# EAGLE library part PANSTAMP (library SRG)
panStamp panStamps are small wireless modules programmable from the Arduino IDE. Each module contains an Atmega328p MCU and a Texas Instruments CC1101 RF interface, providing the necessary connectivity and processing power to create autonomous low-power wireless motes. Everything contained into a compact DIP-24 module. http://www.panstamp.com Vin: 2.5 to 3.6 volts A4 - SDA A5 - SCL PWM: D3,5,6,9,10,11 Interrupts: D2,3
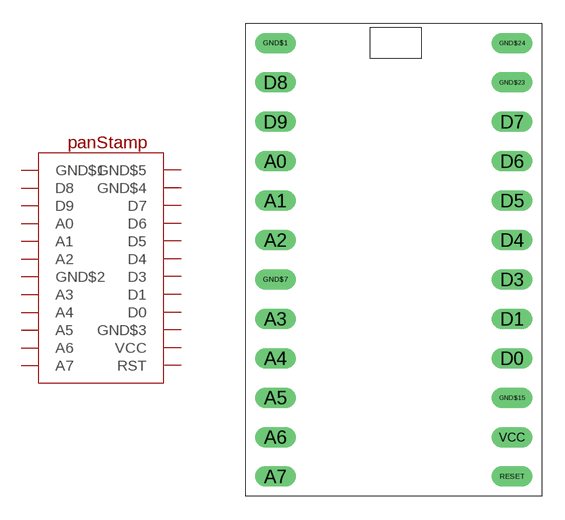
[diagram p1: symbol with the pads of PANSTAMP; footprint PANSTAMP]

Designator prefix -

## PANSTAMP  [PANSTAMP]
A0  A0
A1  A1
A2  A2
A3  A3
A4  A4
A5  A5
A6  A6
A7  A7
D0  D0
D1  D1
D3  D3
D4  D4
D5  D5
D6  D6
D7  D7
D8  D8
D9  D9
GND$1  GND$1  pwr
GND$7  GND$2  pwr
GND$15  GND$3  pwr
GND$23  GND$4  pwr
GND$24  GND$5  pwr
RESET  RST
VCC  VCC  pwr

## Footprint PANSTAMP (pad centres in mm)
panStamp http://www.panstamp.com/ panStamps are small wireless modules programmable from the Arduino IDE. Each module contains an Atmega328p MCU and a Texas Instruments CC1101 RF interface, providing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
drill 0.8 long: A0 -7.62,7.62; A1 -7.62,5.08; A2 -7.62,2.54; A3 -7.62,-2.54; A4 -7.62,-5.08; A5 -7.62,-7.62; A6 -7.62,-10.16; A7 -7.62,-12.7; D0 7.62,-5.08; D1 7.62,-2.54; D3 7.62,0; D4 7.62,2.54; D5 7.62,5.08; D6 7.62,7.62; D7 7.62,10.16; D8 -7.62,12.7; D9 -7.62,10.16; GND$1 -7.62,15.24; GND$7 -7.62,0; GND$15 7.62,-7.62; GND$23 7.62,12.7; GND$24 7.62,15.24; RESET 7.62,-12.7; VCC 7.62,-10.16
